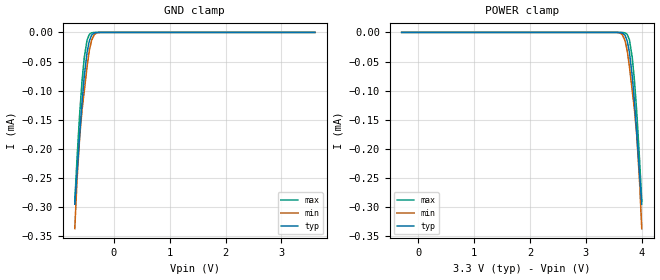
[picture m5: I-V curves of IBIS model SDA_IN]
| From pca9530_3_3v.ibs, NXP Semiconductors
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[Model]   SDA_IN
Model_type Input
Vinh=2.31
Vinl=0.99
C_comp   4p   3.8p   4.2p
[Temperature Range] 27   85   -40
[Voltage Range]   3.3   3   3.6
[GND Clamp]
-700mV    -295uA     -337uA     -289.5uA
-660mV    -241.9uA   -254.1uA   -216.6uA
-610mV    -172.6uA   -176.5uA   -136.3uA
-570mV    -119.6uA   -133.4uA   -83.31uA
-530mV    -75.1uA    -100.5uA   -43.1uA
-480mV    -34.54uA   -59.09uA   -13.06uA
-440mV    -14.75uA   -31.48uA   -3.492uA
-400mV    -4.926uA   -13.83uA   -710.6nA
-350mV    -920.5nA   -3.647uA   -77.68nA
-310mV    -204.4nA   -1.016uA   -12.1nA
-220mV    -5.506nA   -39.51nA   -164pA
3.6V      8.544pA    24.57pA    7.213pA
[POWER Clamp]
-300mV    8.544pA    24.57pA    7.213pA
3.52V     -5.506nA   -39.51nA   -164pA
3.61V     -204.4nA   -1.016uA   -12.1nA
3.65V     -920.5nA   -3.647uA   -77.68nA
3.7V      -4.926uA   -13.83uA   -710.6nA
3.74V     -14.75uA   -31.48uA   -3.492uA
3.78V     -34.54uA   -59.09uA   -13.06uA
3.83V     -75.1uA    -100.5uA   -43.1uA
3.87V     -119.6uA   -133.4uA   -83.31uA
3.91V     -172.6uA   -176.5uA   -136.3uA
3.96V     -241.9uA   -254.1uA   -216.6uA
4V        -295uA     -337uA     -289.5uA
